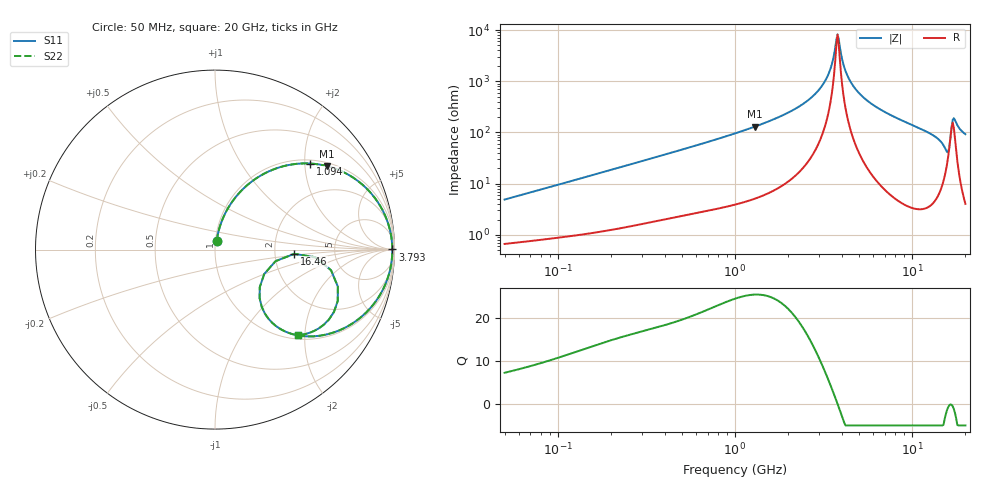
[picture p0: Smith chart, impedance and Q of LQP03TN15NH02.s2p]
!Murata Part Number: LQP03TN15NH02
!These Parameters are Measured in Series Mode Connection
!  o--[Z]--o
!Port1  Port2
!  o-------o
!Freq. Start=50[MHz] Stop=20[GHz], 401[Steps]
# Hz S RI R 50
!Freq.(Hz) S11(Real) S11(Imag) S21(Real) S21(Imag) S12(Real) S12(Imag) S22(Real) S22(Imag)
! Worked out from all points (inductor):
!   401 points, 50 MHz to 20 GHz, reference 50 ohm
!   read as one part in series: L = 15.3 nH near 51.52 MHz
!   highest Q = 25.5 at 1.29 GHz (marker M1), where L = 16 nH
!   self-resonance near 3.793 GHz
!   S11 on the Smith chart (normalised r, x): 50 MHz: 1.01, +0.10; 1.094 GHz: 1.08, +2.12; 3.793 GHz: open; 16.46 GHz: 2.57, -0.15; 20 GHz: 1.08, -1.85
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5e7  0.00894 0.0478  0.9911 -0.0478  0.9911 -0.0478  0.00894 0.0478
1.364002e8  0.0258 0.1237  0.9742 -0.1237  0.9742 -0.1237  0.0258 0.1237
3.721004e8  0.1187 0.2969  0.8813 -0.2969  0.8813 -0.2969  0.1187 0.2969
1e9  0.4798 0.4796  0.5202 -0.4796  0.5202 -0.4796  0.4798 0.4796
1.094034e9  0.5293 0.4796  0.4707 -0.4796  0.4707 -0.4796  0.5293 0.4796
1.289994e9  0.6223 0.4656  0.3777 -0.4656  0.3777 -0.4656  0.6223 0.4656
1.99176e9  0.8444 0.3406  0.1556 -0.3406  0.1556 -0.3406  0.8444 0.3406
2.728004e9  0.9487 0.1877  0.0513 -0.1877  0.0513 -0.1877  0.9487 0.1877
3.314454e9  0.981 0.0788  0.019 -0.0788  0.019 -0.0788  0.981 0.0788
3.792786e9  0.988 0.000582  0.012 -0.000582  0.012 -0.000582  0.988 0.000582
3.908127e9  0.9878 -0.0169  0.0122 0.0169  0.0122 0.0169  0.9878 -0.0169
4.212059e9  0.9846 -0.0607  0.0154 0.0607  0.0154 0.0607  0.9846 -0.0607
4.677679e9  0.9734 -0.1215  0.0266 0.1215  0.0266 0.1215  0.9734 -0.1215
5.683258e9  0.9316 -0.2305  0.0684 0.2305  0.0684 0.2305  0.9316 -0.2305
7.442007e9  0.8286 -0.3631  0.1714 0.3631  0.1714 0.3631  0.8286 -0.3631
1.334722e10  0.4243 -0.4688  0.5757 0.4688  0.5757 0.4688  0.4243 -0.4688
1.460232e10  0.3178 -0.4069  0.6822 0.4069  0.6822 0.4069  0.3178 -0.4069
1.550395e10  0.2486 -0.2708  0.7514 0.2708  0.7514 0.2708  0.2486 -0.2708
1.646126e10  0.4414 -0.0237  0.5586 0.0237  0.5586 0.0237  0.4414 -0.0237
1.747767e10  0.6838 -0.2862  0.3162 0.2862  0.3162 0.2862  0.6838 -0.2862
1.855685e10  0.5755 -0.4407  0.4245 0.4407  0.4245 0.4407  0.5755 -0.4407
2e10  0.4634 -0.4773  0.5366 0.4773  0.5366 0.4773  0.4634 -0.4773
